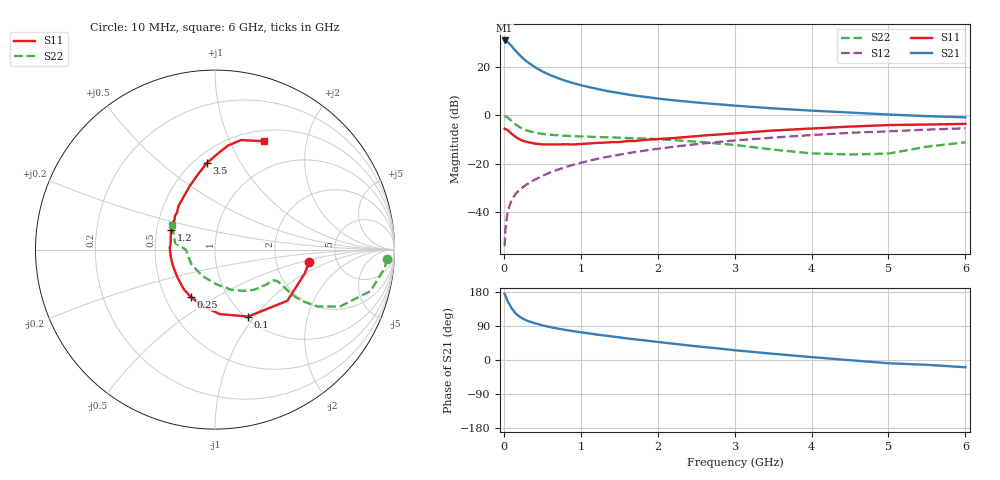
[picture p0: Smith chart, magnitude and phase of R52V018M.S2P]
! SIEMENS Small Signal Semiconductors
! BFR183
! Si NPN RF Bipolar Junction Transistor in SOT23
! VCE = 2 V  IC = 18 mA
! Common Emitter S-Parameters:  May  1996
# GHz  S  MA  R  50
!  f  S11  S21  S12  S22
! GHz  MAG  ANG  MAG  ANG  MAG  ANG  MAG  ANG
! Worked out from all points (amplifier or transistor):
!   36 points, 10 MHz to 6 GHz, reference 50 ohm
!   highest |S21| = 30.8 dB at 10 MHz (marker M1)
!   |S21| within 3 dB of that: start of sweep to 118.7 MHz
!   unconditionally stable (mu >= 1): 541.3 MHz to 2.424 GHz
!   at 250 MHz: K = 0.80, MSG = 26.5 dB, |S12| = -29.6 dB
!   at 1.4 GHz: K = 1.05, MAG = 11.9 dB, |S12| = -16.9 dB
!   at 6 GHz: K = 0.90, MSG = 2.2 dB, |S12| = -5.4 dB
!   S11 on the Smith chart (normalised r, x): 10 MHz: 3.10, -0.61; 100 MHz: 1.03, -0.93; 250 MHz: 0.67, -0.39; 1.2 GHz: 0.59, +0.14; 3.5 GHz: 0.58, +0.72; 6 GHz: 0.63, +1.36
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0.01  0.527 -7.7  34.77 174.8  0.002 88.2  0.9619 -3.0
0.02  0.5184 -14.6  34.57 169.4  0.0044 85.4  0.9499 -6.4
0.05  0.4937 -35.3  32.29 155.5  0.0105 78.6  0.8959 -15.0
0.1  0.4163 -63.6  26.66 137.0  0.0177 70.7  0.7652 -24.5
0.15  0.3604 -85.8  21.53 123.7  0.0237 66.8  0.6538 -29.0
0.2  0.3203 -102.9  17.72 115.2  0.0284 66.4  0.5772 -30.3
0.25  0.2962 -116.8  14.82 108.7  0.0332 66.9  0.5219 -30.5
0.3  0.2819 -127.9  12.73 103.9  0.0378 68.0  0.4845 -29.9
0.4  0.2603 -143.6  9.884 97.3  0.0468 69.1  0.4394 -28.6
0.5  0.2514 -156.9  8.002 91.5  0.056 69.9  0.4119 -27.6
0.6  0.2494 -166.8  6.751 87.0  0.066 70.1  0.3968 -27.1
0.7  0.2495 -174.7  5.845 83.0  0.0753 70.7  0.3857 -27.0
0.8  0.2525 178.0  5.138 79.4  0.085 69.8  0.3766 -27.2
0.9  0.2494 172.2  4.592 76.2  0.095 69.8  0.37 -27.5
1.1  0.2606 161.1  3.822 70.4  0.1144 68.8  0.3616 -29.7
1.2  0.2682 155.6  3.524 67.4  0.1246 68.0  0.3556 -30.6
1.6  0.2926 139.5  2.686 57.0  0.1638 64.3  0.3385 -36.1
2.2  0.3377 122.1  2.034 43.1  0.2234 58.1  0.3085 -46.8
3.5  0.4834 95.6  1.383 16.4  0.3459 41.5  0.1958 -86.2
4.5  0.5832 83.0  1.135 -0.5  0.434 28.6  0.1552 -147.8
5.5  0.6432 70.6  0.956 -12.7  0.5053 16.7  0.2246 170.6
6  0.664 65.5  0.903 -19.2  0.5379 9.0  0.2767 150.3
